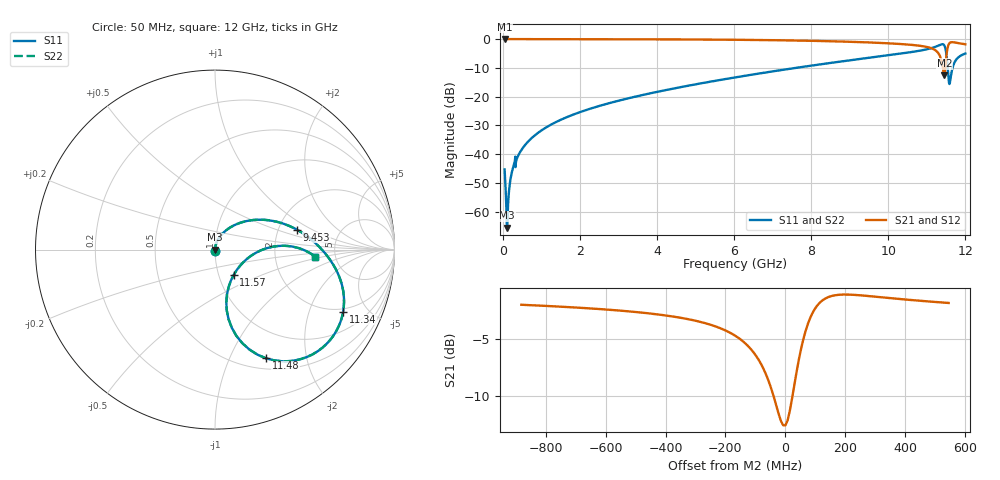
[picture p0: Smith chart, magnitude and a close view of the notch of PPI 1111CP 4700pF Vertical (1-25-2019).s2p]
# GHz S MA R 50
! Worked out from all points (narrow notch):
!   1601 points, 50 MHz to 12 GHz, reference 50 ohm
!   highest |S21| = 0.00 dB at 50 MHz (marker M1); lowest = -12.6 dB at 11.45 GHz (marker M2)
!   notch at M2: 12.4 dB deep, 147 MHz wide at half that depth
!   lowest |S11| = -65.5 dB at 117.2 MHz (marker M3), VSWR 1.00, Z = 50.1 + j0.0161 ohm
!   |S11| at or under -10 dB: start of sweep to 7.603 GHz; 11.54 GHz to 11.67 GHz (124.7 MHz wide, 1.07 % of centre)
!   |S22| runs from -65.5 to -1.8 dB; largest |S21 - S12| = 0
!   S11 on the Smith chart (normalised r, x): 50 MHz: 1.00, -0.01; 9.453 GHz: 2.53, +0.72; 11.34 GHz: 1.84, -3.43; 11.48 GHz: 0.63, -1.38; 11.57 GHz: 1.18, -0.34; 12 GHz: 3.51, -0.41
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0.05  0.00548 -86.1  0.9996 0.0  0.9996 0.0  0.00548 -86.1
0.1172187  0.0005325 17.6  0.9995 -0.6  0.9995 -0.6  0.0005325 17.6
0.1545625  0.001926 72.0  0.9994 -0.9  0.9994 -0.9  0.001926 72.0
0.2068437  0.003824 79.1  0.9993 -1.3  0.9993 -1.3  0.003824 79.1
0.2665938  0.005797 81.1  0.9993 -1.8  0.9993 -1.8  0.005797 81.1
0.5952188  0.01487 82.1  0.9989 -4.1  0.9989 -4.1  0.01487 82.1
1.162844  0.03023 79.4  0.9981 -8.0  0.9981 -8.0  0.03023 79.4
2.044156  0.05509 74.0  0.9966 -14.1  0.9966 -14.1  0.05509 74.0
4.038312  0.1226 60.3  0.9896 -28.5  0.9896 -28.5  0.1226 60.3
6.025  0.2159 45.2  0.9726 -43.9  0.9726 -43.9  0.2159 45.2
8.019156  0.3471 27.9  0.9328 -61.3  0.9328 -61.3  0.3471 27.9
9.453156  0.4691 13.7  0.8767 -75.5  0.8767 -75.5  0.4691 13.7
10.01331  0.5252 7.6  0.8437 -81.7  0.8437 -81.7  0.5252 7.6
10.99172  0.663 -7.2  0.732 -95.8  0.732 -95.8  0.663 -7.2
11.34275  0.7933 -25.9  0.5026 -107.4  0.5026 -107.4  0.7933 -25.9
11.45478  0.7719 -52.5  0.2343 -68.2  0.2343 -68.2  0.7719 -52.5
11.48466  0.6692 -64.8  0.3521 -39.8  0.3521 -39.8  0.6692 -64.8
11.57428  0.1758 -53.9  0.8239 -57.2  0.8239 -57.2  0.1758 -53.9
11.61909  0.217 -6.6  0.8766 -67.8  0.8766 -67.8  0.217 -6.6
11.67884  0.3381 3.1  0.8818 -76.5  0.8818 -76.5  0.3381 3.1
11.79087  0.4631 1.1  0.8557 -85.1  0.8557 -85.1  0.4631 1.1
12  0.5613 -4.1  0.8114 -92.5  0.8114 -92.5  0.5613 -4.1
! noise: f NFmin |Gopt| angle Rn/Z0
0.05  0.0004128  0.8784  0.2719  0.0007345
1.372  0.004378  0.714  7.254  0.003009
2.701  0.007285  0.6731  14.1  0.004231
4.031  0.009974  0.6537  20.73  0.005314
5.36  0.01265  0.6467  27.12  0.006434
6.682  0.01545  0.649  33.22  0.007707
8.012  0.01859  0.6598  39.11  0.009322
9.341  0.02255  0.6814  44.81  0.01178
10.67  0.03232  0.7468  50.94  0.02102
12  0.04189  0.7833  57.2  0.03074
